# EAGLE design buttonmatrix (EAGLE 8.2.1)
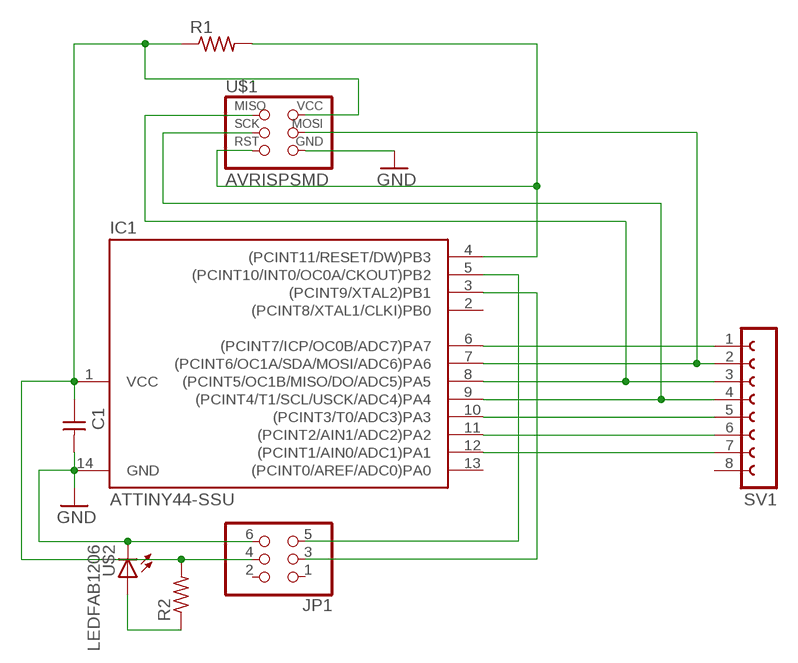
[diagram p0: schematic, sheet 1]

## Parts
C1  CAP-UNPOLARIZEDFAB  [C1206FAB]
IC1  ATTINY44-SSU  [SOIC14]
JP1  PINHD-2X3-SMD  [2X03SMD]
R1  RES-US1206FAB  [R1206FAB]
R2  RES-US1206FAB  [R1206FAB]
SV1  FE08-1  [FE08]
U$1  AVRISPSMD  [2X03SMD]
U$2  LEDFAB1206  [LED1206FAB]

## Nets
GND: C1.2 IC1.14(GND) JP1.6 U$1.6(GND) U$2.2(C)
N$1: IC1.4((PCINT11/RESET/DW)PB3) R1.2 U$1.5(RST)
N$2: IC1.6((PCINT7/ICP/OC0B/ADC7)PA7) SV1.1
N$3: IC1.8((PCINT5/OC1B/MISO/DO/ADC5)PA5) SV1.3 U$1.1(MISO)
N$4: IC1.7((PCINT6/OC1A/SDA/MOSI/ADC6)PA6) SV1.2 U$1.4(MOSI)
N$5: IC1.9((PCINT4/T1/SCL/USCK/ADC4)PA4) SV1.4 U$1.3(SCK)
N$6: IC1.10((PCINT3/T0/ADC3)PA3) SV1.5
N$7: IC1.11((PCINT2/AIN1/ADC2)PA2) SV1.6
N$8: IC1.12((PCINT1/AIN0/ADC1)PA1) SV1.7
N$9: IC1.5((PCINT10/INT0/OC0A/CKOUT)PB2) JP1.5
N$10: IC1.3((PCINT9/XTAL2)PB1) JP1.3
N$12: C1.1 IC1.1(VCC) JP1.4 R1.1 R2.2 U$1.2(VCC)
N$13: R2.1 U$2.1(A)
Unconnected: IC1.2((PCINT8/XTAL1/CLKI)PB0) IC1.13((PCINT0/AREF/ADC0)PA0) JP1.1 JP1.2 SV1.8

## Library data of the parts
C1 = fab:CAP-UNPOLARIZED
IC1 = fab:ATTINY44
JP1 = fab:PINHD-2X3-SMD: PIN HEADER
R1 R2 = fab:RES-US: Resistor (US Symbol)
SV1 = con-lsta:FE08-1: FEMALE HEADER; OC_FARNELL: unknown; OC_NEWARK: unknown
U$1 = fab:AVRISP
U$2 = fab:LED: LED

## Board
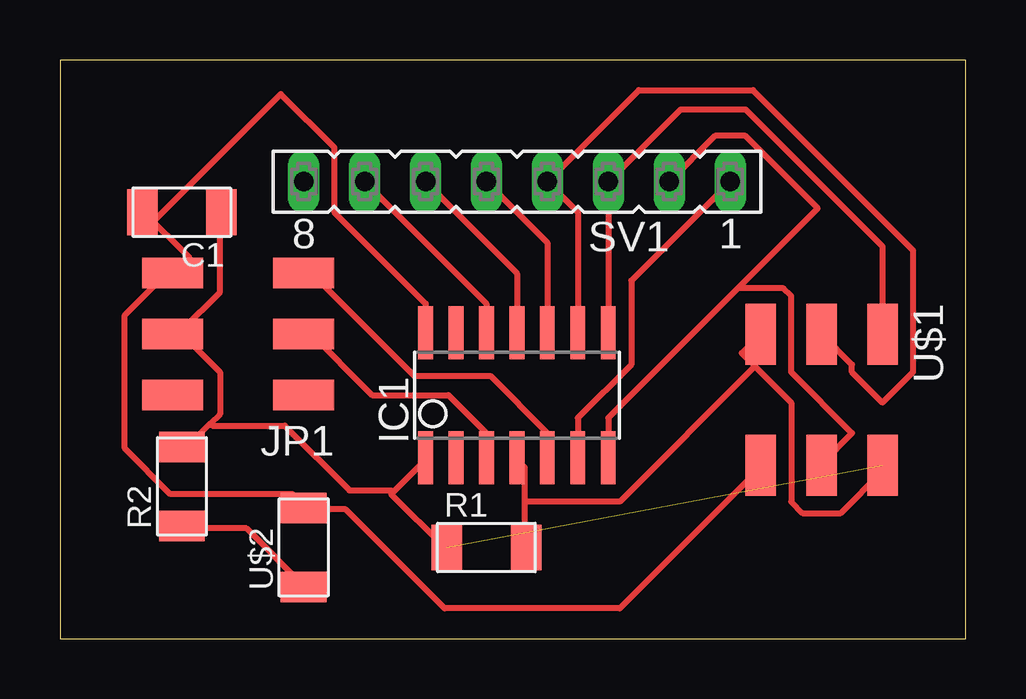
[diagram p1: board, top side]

Size 37.77 x 24.12 mm. Coordinates in mm from the lower left corner, seen from the top.
Outline: 0,0 37.77,0 37.77,24.12 0,24.12 0,0
Copper layers (1*16): Top 0.035mm / dielectric 1.5mm / Bottom 0.035mm
Design rules "default *": minimum track width 10mil, minimum drill 24mil, track to track 18mil, track to pad 18mil, pad to pad 18mil, via to via 18mil, smd to smd 18mil, copper to edge 40mil, drill to drill 8mil, minimum pad ring 10mil, minimum via ring 8mil, stop-mask expansion 4mil, vias tented up to drill 0mil, thermal gap 10mil

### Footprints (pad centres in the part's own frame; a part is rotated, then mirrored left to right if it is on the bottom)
C1206FAB = smd 1.27 x 1.905: 1 -1.651,0; 2 1.651,0
SOIC14 = smd 0.61 x 2.21: 1 -3.81,-2.603; 2 -2.54,-2.603; 3 -1.27,-2.603; 4 0,-2.603; 5 1.27,-2.603; 6 2.54,-2.603; 7 3.81,-2.603; 8 3.81,2.603; 9 2.54,2.603; 10 1.27,2.603; 11 0,2.603; 12 -1.27,2.603; 13 -2.54,2.603; 14 -3.81,2.603
2X03SMD = smd 2.54 x 1.27: 1 -2.54,2.54; 2 2.92,2.54; 3 -2.54,0; 4 2.92,0; 5 -2.54,-2.54; 6 2.92,-2.54
R1206FAB = smd 1.27 x 1.905: 1 -1.651,0; 2 1.651,0
FE08 = drill 0.813 long: 1 -8.89,0; 2 -6.35,0; 3 -3.81,0; 4 -1.27,0; 5 1.27,0; 6 3.81,0; 7 6.35,0; 8 8.89,0
LED1206FAB = smd 1.27 x 1.905: 1 -1.651,0; 2 1.651,0

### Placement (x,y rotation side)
C1  5.08,17.78 180 top
IC1  19.05,10.16 0 top
JP1  7.62,12.7 180 top
R1  17.78,3.81 0 top
R2  5.08,6.35 90 top
SV1  19.05,19.05 180 top
U$1  31.75,10.16 270 top
U$2  10.16,3.81 90 top

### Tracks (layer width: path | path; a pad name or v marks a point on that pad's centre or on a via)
GND
  Top 0.254: IC1.14 15.24,13.97 11.43,17.78 11.43,20.48 9.21,22.7 3.97,17.46 C1.2 3.49,17.78 5.4,15.88 4.76,15.24 JP1.6 4.45,15.24 2.7,13.49 2.7,7.94 4.6,6.03 9.68,6.03 10.16,5.56 U$2.2 10.16,5.4 11.91,5.4 16.03,1.27 23.34,1.27 29.21,7.14 U$1.6
N$1
  Top 0.254: 19.37,5.71 19.37,7.14 19.05,7.46 IC1.4 | 19.37,5.71 19.37,3.81 R1.2 | 34.29,6.99 32.54,5.24 30.96,5.24 30.48,5.71 30.48,9.84 28.97,11.35 | 28.97,11.35 28.42,11.91 U$1.5 | 19.37,5.71 23.34,5.71 28.97,11.35
N$2
  Top 0.254: IC1.6 21.59,9.21 23.81,11.43 23.81,14.92 SV1.1
N$3
  Top 0.254: IC1.8 SV1.3 25.88,22.07 28.57,22.07 34.29,16.35 U$1.1
N$4
  Top 0.254: IC1.7 22.86,9.21 28.26,14.61 | 28.26,14.61 30.16,14.61 30.48,14.29 30.48,11.11 33.02,8.57 31.75,7.3 U$1.4 | SV1.2 27.3,20.95 28.57,20.95 31.59,17.94 28.26,14.61
N$5
  Top 0.254: IC1.9 21.59,17.78 SV1.4 24.13,22.86 28.89,22.86 35.56,16.19 35.56,11.11 34.29,9.84 33.02,11.11 33.02,11.43 U$1.3
N$6
  Top 0.254: IC1.10 20.32,16.51 SV1.5
N$7
  Top 0.254: IC1.11 19.05,15.24 SV1.6
N$8
  Top 0.254: IC1.12 17.78,13.97 SV1.7
N$9
  Top 0.254: IC1.5 20.32,8.57 17.94,10.95 14.76,10.95 10.32,15.4 JP1.5
N$10
  Top 0.254: IC1.3 17.78,8.57 16.19,10.16 13.02,10.16 10.32,12.86 JP1.3
N$12  (1 unrouted)
  Top 0.254: 13.89,6.11 15.24,7.46 IC1.1 | 13.89,6.11 13.81,6.03 16.03,3.81 R1.1 | 6.27,8.97 6.67,9.37 6.67,11.11 4.92,12.86 4.76,12.7 JP1.4 5.08,12.86 6.67,14.45 6.67,17.78 C1.1 | 6.27,8.97 5.4,8.1 5.08,8.1 R2.2 | 13.89,6.11 13.81,6.19 12.06,6.19 9.37,8.89 6.35,8.89 6.27,8.97
N$13
  Top 0.254: R2.1 5.08,4.6 7.78,4.6 10.16,2.22 U$2.1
